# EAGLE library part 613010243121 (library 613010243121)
WR-PHD 2.54 mm Socket Header 10p 2 rows Right angle Source: Datasheet
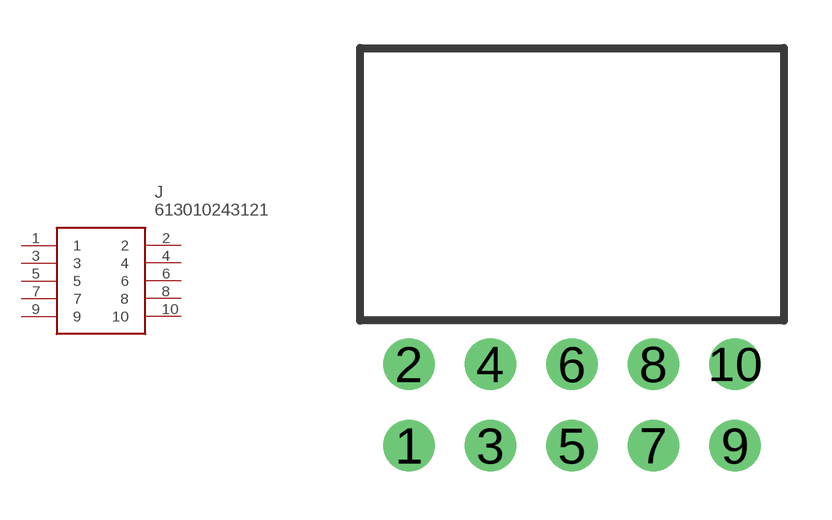
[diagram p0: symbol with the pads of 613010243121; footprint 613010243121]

Designator prefix J

## 613010243121 (Description: WR-PHD 2.54 mm Socket Header 10p 2 rows Right angle; Height: mm; Manufacturer_Name: Wurth Elektronik; Manufacturer_Part_Number: 613010243121; Mouser_Part_Number: 710-613010243121; Mouser_Price-Stock: https://www.mouser.co.uk/ProductDetail/Wurth-Elektronik/613010243121?qs=ZtY9WdtwX54mDpZwGjr8IA%3D%3D)  [613010243121]
1  1
2  2
3  3
4  4
5  5
6  6
7  7
8  8
9  9
10  10

## Footprint 613010243121 (pad centres in mm)
613010243121
drill 1.07 pad 1.6: 1 -5.08,-12.4; 2 -5.08,-9.86; 3 -2.54,-12.4; 4 -2.54,-9.86; 5 0,-12.4; 6 0,-9.86; 7 2.54,-12.4; 8 2.54,-9.86; 9 5.08,-12.4; 10 5.08,-9.86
